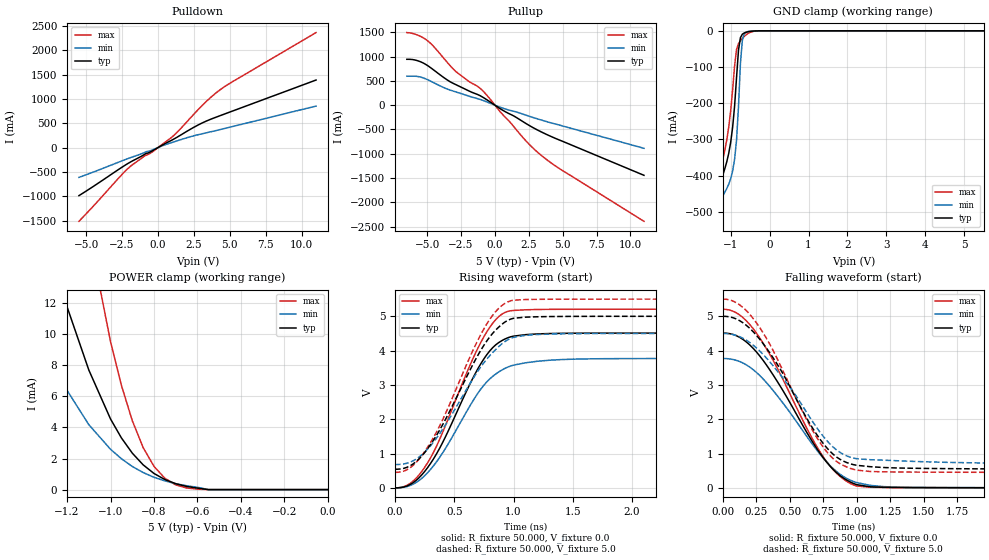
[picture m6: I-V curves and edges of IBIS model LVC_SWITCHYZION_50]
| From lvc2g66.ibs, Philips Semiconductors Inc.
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|   Model LVC_SWITCHYZION_50
[Model]   LVC_SWITCHYZION_50
Model_type   I/O
Polarity   Non-Inverting
Enable   Active-High
Vinl  =  1.5V
Vinh  =  3.5V
Vmeas =  2.5V
Cref  =  50.0pF
Rref  =  0.5k
Vref  =  0.0V
C_comp   7.71pF   4.34pF   10.52pF
[Model Spec]
| Note: The input and output voltage ratings may be exceeded if the input and
|   output current ratings are observed (please refer to the data sheet)
|   Subparameter   typ   min   max
| Thresholds
Vinh   3.5   3.15   3.85
Vinl   1.5   1.35   1.65
| Overshoot
S_overshoot_high   6.5   6.5   6.5   | Static overshoot
S_overshoot_low   -0.5   -0.5   -0.5
D_overshoot_high   11.0   11.0   11.0   | Dynamic overshoot
D_overshoot_low   -0.95   -0.9   -1.0
D_overshoot_time   3n   3n   3n
| Timing Thresholds
Vmeas   2.5   2.25   2.75
|Ambient temperature:   25   85   -40
[Temperature Range]   50   105   -10
[Voltage Range]   5.0V   4.5V   5.5V
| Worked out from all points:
|   slope of the pulldown table from 0 to 0.75 V, typ, clamps not added: 6.21 ohm
|   slope of the pullup table from 0 to 0.75 V, typ, clamps not added: 5.68 ohm
|   GND clamp passes 1 mA (typ) near -0.44 V on its own axis
|   POWER clamp passes 1 mA (typ) near -0.80 V on its own axis
|   rising waveform, R_fixture 50.000, V_fixture 0.0: 20-80 % time 388ps typ, 407ps min, 387ps max; typ from 0 V to 4.51 V
|   rising waveform, R_fixture 50.000, V_fixture 5.0: 20-80 % time 409ps typ, 422ps min, 403ps max; typ from 0.542 V to 5 V
|   falling waveform, R_fixture 50.000, V_fixture 0.0: 20-80 % time 425ps typ, 439ps min, 419ps max; typ from 4.51 V to 0 V
|   falling waveform, R_fixture 50.000, V_fixture 5.0: 20-80 % time 404ps typ, 426ps min, 398ps max; typ from 5 V to 0.542 V
|Process Range   nominal   slow   fast
[Pulldown]
| voltage   I(typ)   I(min)   I(max)
-5.5V     -988.3mA   -613.1mA   -1.516A
-2.1V     -328.4mA   -226.9mA   -433.1mA
-950mV    -142.5mA   -102.8mA   -176.1mA
-400mV    -67.79mA   -48.85mA   -89.77mA
1V        158.6mA    107.1mA    222.5mA
2.8V      465.9mA    265.4mA    782.5mA
4V        620.9mA    347.6mA    1.116A
5.2V      753.2mA    434.2mA    1.358A
11V       1.39A      854.2mA    2.366A
[Pullup]
| voltage   I(typ)   I(min)   I(max)
-6.5V     944.7mA    596.6mA    1.495A
-5.9V     930.3mA    596.6mA    1.463A
-5.1V     838.3mA    540.6mA    1.354A
-4.5V     720.5mA    459.9mA    1.202A
-3.5V     516.1mA    330.1mA    876mA
-2.9V     425mA      274.4mA    696.7mA
-1.1V     196.6mA    119.2mA    349.2mA
600mV     -108.5mA   -63.45mA   -201.6mA
2.2V      -361.9mA   -196.9mA   -708.2mA
3.6V      -574.8mA   -320.9mA   -1.074A
4.8V      -722.5mA   -413.3mA   -1.313A
11V       -1.444A    -887.9mA   -2.391A
[GND_clamp]
| voltage   I(typ)   I(min)   I(max)
-5.5V     -4.658A    -4.678A    -4.682A
-1.45V    -594.6mA   -645.1mA   -560mA
-1.35V    -501.1mA   -552.3mA   -465.3mA
-1.25V    -420.3mA   -474mA     -381.5mA
-1.05V    -338.5mA   -424mA     -265.6mA
-900mV    -208.1mA   -355.1mA   -97.15mA
-850mV    -129.6mA   -302.2mA   -51.89mA
-800mV    -53.65mA   -210.5mA   -35.41mA
-750mV    -18.9mA    -90.02mA   -27.35mA
-700mV    -9.267mA   -25.77mA   -20.97mA
-600mV    -3.924mA   -3.148mA   -10.77mA
5.5V      6.381nA    27.55nA    3.404nA
[POWER_clamp]
| voltage   I(typ)   I(min)   I(max)
-6.5V     4.731A     4.763A     4.744A
-1.4V     22.5mA     17.16mA    47.34mA
-1.3V     16.65mA    9.878mA    35.79mA
-1.2V     11.77mA    6.39mA     25.47mA
-1.1V     7.702mA    4.182mA    16.62mA
-1V       4.546mA    2.596mA    9.523mA
-950mV    3.329mA    1.988mA    6.715mA
-900mV    2.349mA    1.492mA    4.439mA
-850mV    1.594mA    1.098mA    2.706mA
-750mV    647.2uA    559.6uA    730uA
-600mV    95.32uA    150uA      30.97uA
0V        0A         0A         0A
[Ramp]
| variable   typ   min   max
dV/dt_r   2.706V/387.524ps   2.262V/406.622ps   3.123V/387.075ps
dV/dt_f   2.675V/404.130ps   2.293V/426.405ps   3.029V/398.365ps
R_load = 50.000
[Rising Waveform]
R_fixture   = 50.000
V_fixture   = 0.0
V_fixture_min = 0.0
V_fixture_max = 0.0
| time   V(typ)   V(min)   V(max)
0s        883.9fV    21.88pV    43.15fV
125ps     91.86mV    64mV       123.4mV
250ps     476.3mV    352.3mV    596.3mV
375ps     1.144V     879.1mV    1.402V
625ps     2.977V     2.348V     3.514V
750ps     3.76V      2.993V     4.405V
875ps     4.234V     3.378V     4.99V
975ps     4.401V     3.551V     5.16V
1.8ns     4.509V     3.765V     5.205V
8.8ns     4.511V     3.77V      5.205V
[Rising Waveform]
R_fixture   = 50.000
V_fixture   = 5.0
V_fixture_min = 4.5
V_fixture_max = 5.5
| time   V(typ)   V(min)   V(max)
0s        542.1mV    678.4mV    451.4mV
125ps     637.7mV    745.4mV    578.6mV
250ps     1.027V     1.04V      1.053V
400ps     1.828V     1.698V     1.971V
650ps     3.549V     3.137V     3.95V
750ps     4.156V     3.648V     4.635V
875ps     4.685V     4.118V     5.232V
1ns       4.942V     4.386V     5.47V
1.7ns     4.999V     4.497V     5.499V
8.8ns     5V         4.5V       5.5V
[Falling Waveform]
R_fixture   = 50.000
V_fixture   = 0.0
V_fixture_min = 0.0
V_fixture_max = 0.0
| time   V(typ)   V(min)   V(max)
0s        4.511V     3.77V      5.205V
100ps     4.435V     3.716V     5.102V
225ps     4.071V     3.448V     4.645V
375ps     3.293V     2.839V     3.72V
625ps     1.63V      1.51V      1.753V
750ps     878.7mV    867mV      905mV
875ps     359.2mV    398.3mV    337.5mV
1ns       93.48mV    154.2mV    54.42mV
1.5ns     7.622mV    10.34mV    5.422mV
8.8ns     4.679uV    73.72uV    95.16nV
[Falling Waveform]
R_fixture   = 50.000
V_fixture   = 5.0
V_fixture_min = 4.5
V_fixture_max = 5.5
| time   V(typ)   V(min)   V(max)
0s        5V         4.5V       5.5V
125ps     4.872V     4.406V     5.333V
275ps     4.333V     3.989V     4.671V
425ps     3.485V     3.317V     3.607V
650ps     1.871V     2.053V     1.817V
775ps     1.174V     1.385V     1.058V
875ps     832.7mV    1.035V     704.4mV
1ns       657.6mV    849.5mV    516.1mV
2.7ns     545.6mV    698.8mV    451.8mV
8.8ns     542.1mV    678.5mV    451.4mV
